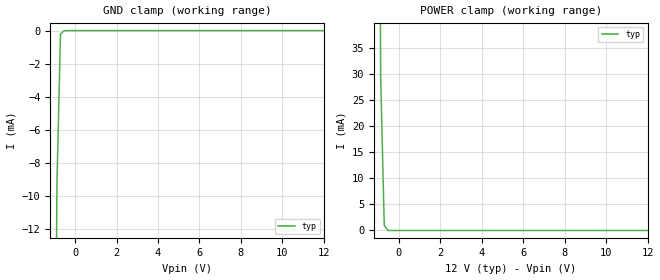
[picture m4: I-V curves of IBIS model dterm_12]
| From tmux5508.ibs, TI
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| dterm_12
[Model]   dterm_12
Model_type   Terminator
|   typ   min   max
C_comp   6.362683e-12   NA   NA
[Voltage Range]   12   NA   NA
[Temperature Range]   27   NA   NA
[Power Clamp Reference]   12   NA   NA
[GND Clamp Reference]   0   NA   NA
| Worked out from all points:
|   GND clamp passes 1 mA (typ) near -0.72 V on its own axis
|   POWER clamp passes 1 mA (typ) near -0.70 V on its own axis
[GND Clamp]
|   Voltage   I(typ)   I(min)   I(max)
-5V       -2.839A    NA         NA
-1.051V   -42.72mA   NA         NA
-878.8mV  -9.288mA   NA         NA
-707.1mV  -223.6uA   NA         NA
-535.4mV  -9.048uA   NA         NA
12V       1.089nA    NA         NA
[POWER Clamp]
|   Voltage   I(typ)   I(min)   I(max)
-5V       8.448A     NA         NA
-1.05V    167.3mA    NA         NA
-878.8mV  29.56mA    NA         NA
-707.1mV  1.029mA    NA         NA
-535.4mV  6.118uA    NA         NA
12V       -1.319nA   NA         NA
